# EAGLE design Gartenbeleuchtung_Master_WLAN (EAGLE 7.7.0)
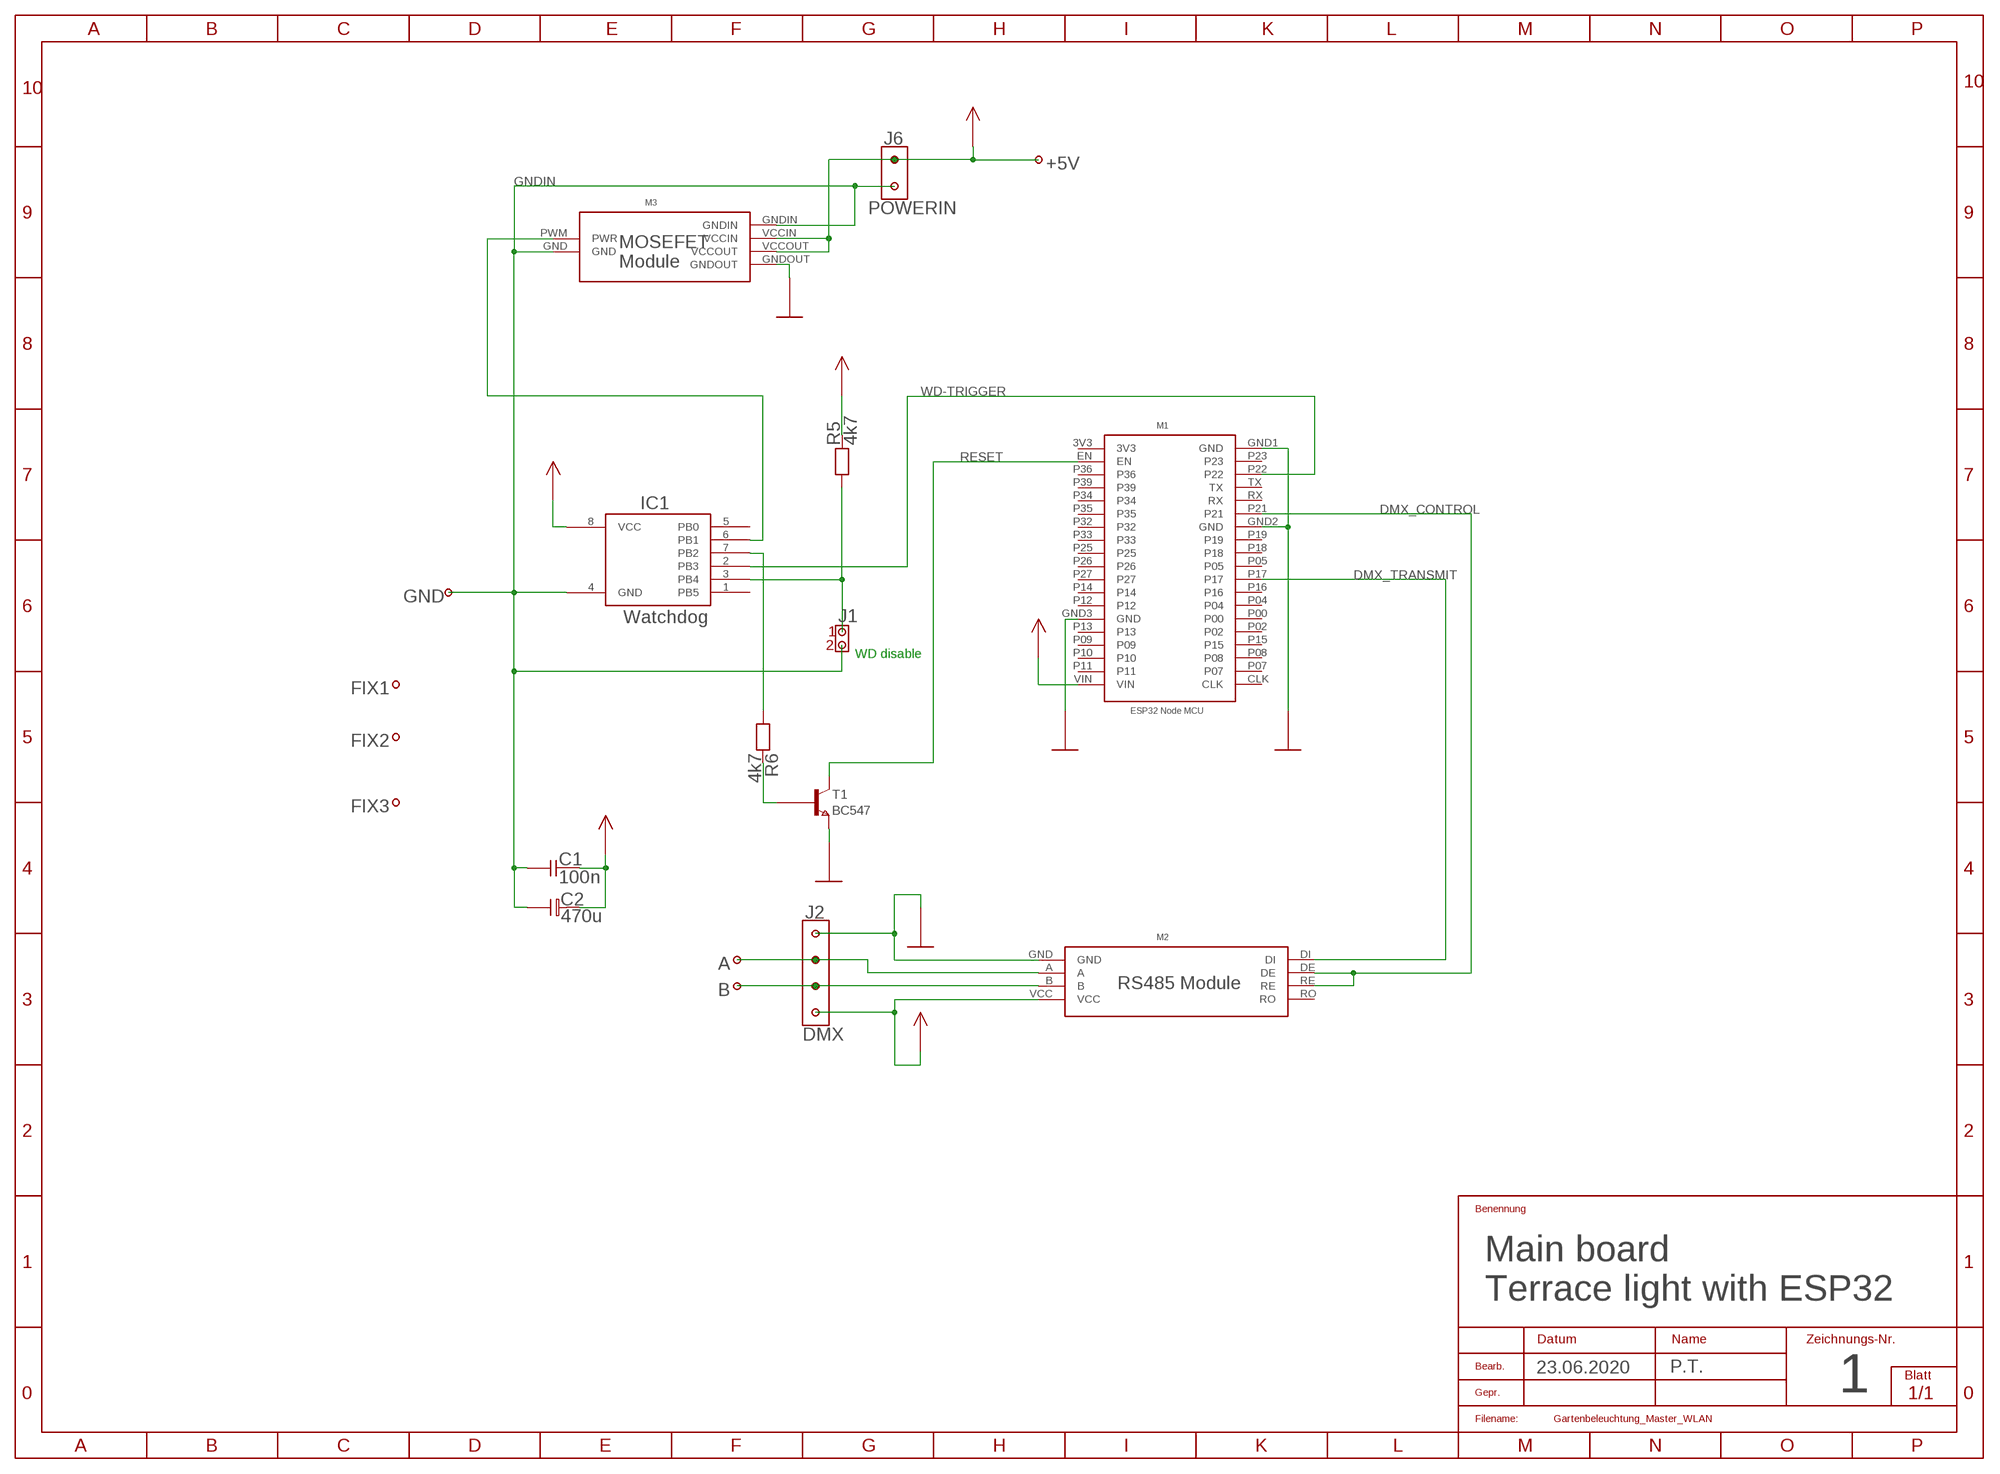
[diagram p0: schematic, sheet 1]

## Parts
+5V  PIN  [PIN]
A  PIN  [PIN]
B  PIN  [PIN]
C1  100n  CAP02  [CAP02B]
C2  470u  ELK02LI  [ELKOL02B]
FIX1  PIN  [PIN]
FIX2  PIN  [PIN]
FIX3  PIN  [PIN]
GND  PIN  [PIN]
IC1  Watchdog  ATINY13A  [DIL8]
J1  WD disable  CON02X1  [CON02X1]
J2  DMX  POWER4X1  [POWER4X1]
J6  POWERIN  POWER2X1  [POWER2X1]
M1  ESP32-NODEMCU1  [ESP32-NODEMCU1]
M2  RS485  [RS485]
M3  MOSFET  [MOSFET]
R5  4k7  RES04  [RES04B]
R6  4k7  RES04  [RES04B]
T1  BC547  BC237  [TO92A]

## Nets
DMX_CONTROL: M1.P21 M2.DE M2.RE
DMX_TRANSMIT: M1.P17 M2.DI
GND: J2.4 M1.GND1(GND) M1.GND2(GND) M1.GND3(GND) M2.GND M3.GNDOUT T1.3(E)
GNDIN: C1.1 C2.N GND.1 IC1.4(GND) J1.2 J6.1 M3.GND M3.GNDIN
N$4: IC1.3(PB4) J1.1 R5.1
N$5: A.1 J2.3 M2.A
N$6: B.1 J2.2 M2.B
N$7: IC1.7(PB2) R6.1
N$8: IC1.6(PB1) M3.PWM(PWR)
N$9: R6.2 T1.2(B)
RESET: M1.EN T1.1(C)
VCC: +5V.1 C1.2 C2.P IC1.8(VCC) J2.1 J6.2 M1.VIN M2.VCC M3.VCCIN M3.VCCOUT R5.2
WD-TRIGGER: IC1.2(PB3) M1.P22
Unconnected: FIX1.1 FIX2.1 FIX3.1 IC1.1(PB5) IC1.5(PB0) M1.CLK M1.P00 M1.P02 M1.P04 M1.P05 M1.P07 M1.P08 M1.P09 M1.P10 M1.P11 M1.P12 M1.P13 M1.P14 M1.P15 M1.P16 M1.P18 M1.P19 M1.P23 M1.P25 M1.P26 M1.P27 M1.P32 M1.P33 M1.P34 M1.P35 M1.P36 M1.P39 M1.RX M1.TX M2.RO

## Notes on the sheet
- WD disable
- Main board
- Terrace light with ESP32
- 23.06.2020 | P.T.
- 1

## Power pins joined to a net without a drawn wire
3V3: M1.3V3

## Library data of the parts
+5V A B FIX1-FIX3 GND = Connector 2:PIN
C1 = Discrete:CAP02
C2 = Discrete:ELK02LI
IC1 = Processor:ATINY13A
J1 = Connector 1:CON02X1
J2 = Connector 2:POWER4X1
J6 = Connector 2:POWER2X1
M1 = Giess:ESP32-NODEMCU1
M2 = Giess:RS485
M3 = Giess:MOSFET
R5 R6 = Discrete:RES04
T1 = Transistor:BC237

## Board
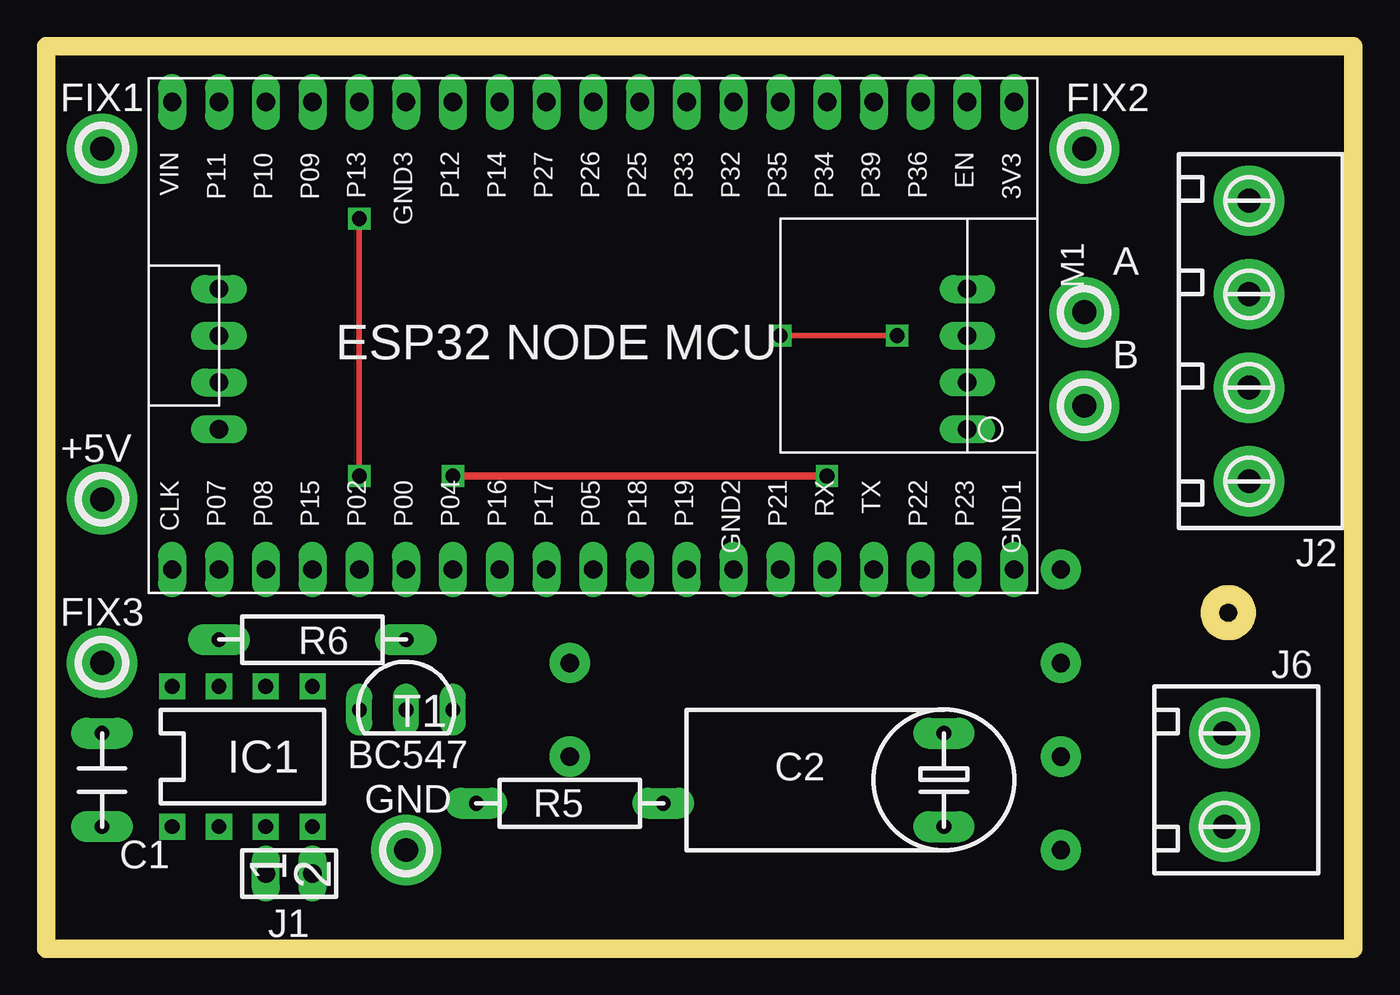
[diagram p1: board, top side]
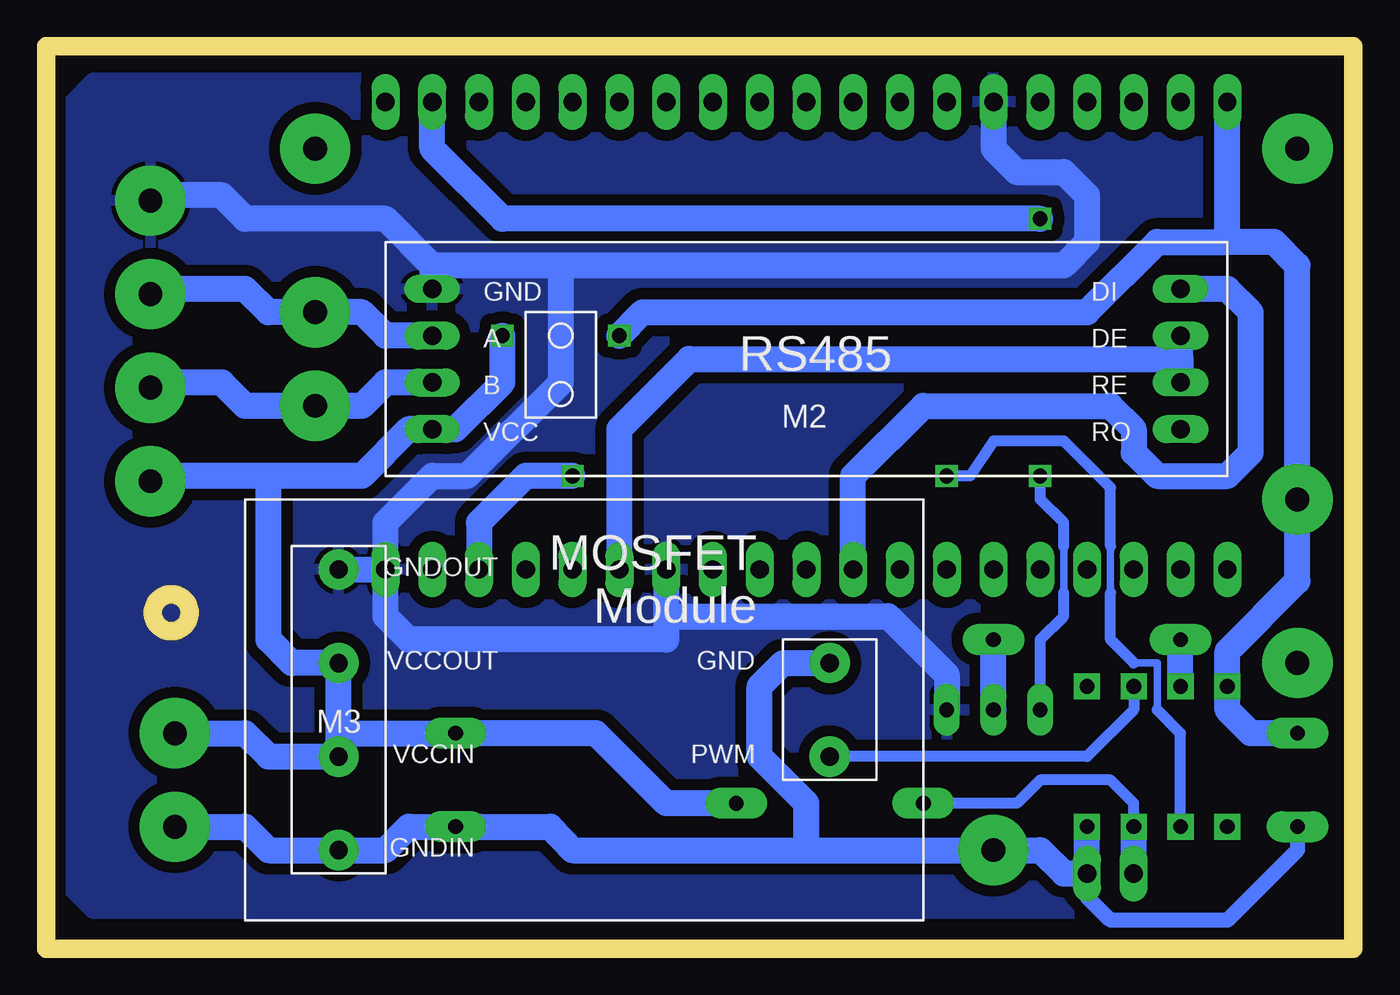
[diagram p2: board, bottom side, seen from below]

Size 71 x 49.04 mm. Coordinates in mm from the lower left corner, seen from the top.
Outline: 0,49.04 71,49.04 71,0 0,0 0,49.04
Copper layers (1*16): Top 0.035mm / dielectric 1.5mm / Bottom 0.035mm
Design rules "default": minimum track width 10mil, minimum drill 24mil, track to track 8mil, track to pad 8mil, pad to pad 8mil, via to via 8mil, smd to smd 8mil, copper to edge 40mil, drill to drill 8mil, minimum pad ring 10mil, minimum via ring 8mil, stop-mask expansion 4mil, vias tented up to drill 0mil, thermal gap 10mil
Milling: 6 lines

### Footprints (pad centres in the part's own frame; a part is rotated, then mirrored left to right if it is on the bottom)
PIN = drill 1.3 pad 3.81: 1 0,0
CAP02B = drill 0.8 pad 1.676 long: 1 0,0; 2 5.08,0
ELKOL02B = drill 0.8 pad 1.676 long: N 5.08,0; P 0,0
DIL8 = drill 0.8 pad 1.422 square: 1 0,0; 2 2.54,0; 3 5.08,0; 4 7.62,0; 5 7.62,7.62; 6 5.08,7.62; 7 2.54,7.62; 8 0,7.62
CON02X1 = drill 1 pad 1.422 long: 1 0,0; 2 0,-2.54
POWER4X1 = drill 1.3 pad 3.81: 1 0,0; 2 0,5.08; 3 0,10.16; 4 0,15.24
POWER2X1 = drill 1.3 pad 3.81: 1 0,0; 2 0,5.08
ESP32-NODEMCU1 = drill 1 pad 1.422 long: 3V3 -22.86,-12.7; CLK 22.86,12.7; EN -20.32,-12.7; GND1 -22.86,12.7; GND2 -7.62,12.7; GND3 10.16,-12.7; P00 10.16,12.7; P02 12.7,12.7; P04 7.62,12.7; P05 0,12.7; P07 20.32,12.7; P08 17.78,12.7; P09 15.24,-12.7; P10 17.78,-12.7; P11 20.32,-12.7; P12 7.62,-12.7; P13 12.7,-12.7; P14 5.08,-12.7; P15 15.24,12.7; P16 5.08,12.7; P17 2.54,12.7; P18 -2.54,12.7; P19 -5.08,12.7; P21 -10.16,12.7; P22 -17.78,12.7; P23 -20.32,12.7; P25 -2.54,-12.7; P26 0,-12.7; P27 2.54,-12.7; P32 -7.62,-12.7; P33 -5.08,-12.7; P34 -12.7,-12.7; P35 -10.16,-12.7; P36 -17.78,-12.7; P39 -15.24,-12.7; RX -12.7,12.7; TX -15.24,12.7; VIN 22.86,-12.7
RS485 = drill 1 pad 1.422 long: A -20.32,0; B -20.32,-2.54; DE 20.32,0; DI 20.32,2.54; GND -20.32,2.54; RE 20.32,-2.54; RO 20.32,-5.08; VCC -20.32,-5.08
MOSFET = drill 1 pad 2.184: GND -19.05,-5.08; GNDIN 7.62,5.08; GNDOUT 7.62,-10.16; PWM -19.05,0; VCCIN 7.62,0; VCCOUT 7.62,-5.08
RES04B = drill 0.8 pad 1.676 long: 1 0,0; 2 10.16,0
TO92A = drill 0.8 pad 1.422 long: 1 0,0; 2 2.54,0; 3 5.08,0

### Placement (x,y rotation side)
+5V  3.04,24.42 0 top
A  56.38,34.58 0 top
B  56.38,29.5 0 top
C1  3.04,6.64 90 top
C2  48.76,11.72 270 top
FIX1  3.04,43.47 0 top
FIX2  56.38,43.47 0 top
FIX3  3.04,15.53 0 top
GND  19.55,5.37 0 top
IC1  6.85,6.64 0 top
J1  11.93,4.1 90 top
J2  65.33,25.4 0 top
J6  64,6.64 0 top
M1  29.71,33.31 180 top
M2  29.71,33.31 0 bottom
M3  47.49,10.45 180 bottom
R5  23.36,7.91 0 top
R6  9.39,16.8 0 top
T1  17.01,12.99 0 top

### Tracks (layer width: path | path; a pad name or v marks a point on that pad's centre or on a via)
DMX_CONTROL
  Bottom 1.422: M1.P21 39.87,28.23 36.06,32.04 9.39,32.04 | 9.39,32.04 M2.RE | 9.39,32.04 M2.DE
DMX_TRANSMIT
  Bottom 1.422: M1.P17 27.17,25.69 23.36,29.5 13.2,29.5 11.93,28.23 11.93,26.96 10.66,25.69 6.85,25.69 5.58,26.96 5.58,34.58 6.85,35.85 M2.DI
GND
  Bottom 1.422: M3.GNDOUT M1.GND1 | 37.33,18.07 37.33,16.8 51.3,16.8 52.57,18.07 M1.GND1 | M1.GND2 37.33,18.07 | 37.33,18.07 25.27,18.07 22.09,14.9 T1.3 | M1.GND3 19.55,43.47 18.28,42.2 15.74,42.2 14.47,40.93 14.47,38.39 15.74,37.12 43.05,37.12 | 50.03,37.12 52.57,39.66 60.19,39.66 61.46,40.93 65.04,40.93 J2.4 | M1.GND1 52.57,23.15 50.03,25.69 48.12,25.69 43.05,30.77 43.05,37.12 | 43.05,37.12 50.03,37.12 | 50.03,37.12 M2.GND
  pour Bottom (isolate 0.61): 5.83,47.28 68.51,47.28 69.84,45.95 69.84,3.27 68.51,1.94 1.83,1.94 0.5,3.27 0.5,45.95 1.83,47.28
GNDIN
  Bottom 0.813: C1.1 3.04,5.37 6.85,1.56 13.2,1.56 14.47,2.83 J1.2
  Bottom 1.422: J6.1 60.19,6.64 58.92,5.37 M3.GNDIN 52.57,5.37 51.3,6.64 C2.N | 47.49,6.64 C2.N | C2.N 43.62,6.64 42.41,5.37 29.71,5.37 | 29.71,5.37 29.71,7.91 32.25,10.45 32.25,14.26 30.98,15.53 M3.GND | IC1.4 J1.2 15.74,4.1 17.01,5.37 GND.1 29.71,5.37
N$4
  Bottom 0.61: IC1.3 11.93,7.91 13.2,9.18 17.01,9.18 18.28,7.91 R5.1
  Bottom 1.422: J1.1 IC1.3
N$5
  Bottom 1.422: M2.A 52.57,33.31 53.84,34.58 A.1 58.92,34.58 60.19,35.85 65.04,35.85 J2.3
N$6
  Bottom 1.422: M2.B 52.57,30.77 53.84,29.5 B.1 60.19,29.5 61.46,30.77 65.27,30.77 65.27,30.54 J2.2
N$7
  Bottom 1.422: IC1.7 R6.1
N$8
  Bottom 0.61: IC1.6 11.93,12.99 14.47,10.45 M3.PWM
N$9
  Bottom 1.422: T1.2 R6.2
RESET  (via drill 0.8 pad 0.61, 0.8 pad 0.81)
  Top 0.305: v17.01,25.69 v17.01,39.66
  Bottom 0.406: 15.74,19.34 15.74,21.88
  Bottom 0.61: T1.1 17.01,16.8 15.74,18.07 15.74,19.34 | 15.74,21.88 15.74,23.15 17.01,24.42 v17.01,25.69
  Bottom 1.422: v17.01,39.66 46.22,39.66 50.03,43.47 M1.EN
VCC  (via drill 0.8 pad 0.81)
  Top 0.305: v46.22,33.31 v39.87,33.31
  Bottom 1.422: J6.2 60.19,11.72 58.92,10.45 M3.VCCIN | M3.VCCIN M3.VCCOUT 57.65,15.53 58.92,16.8 58.92,25.69 | M3.VCCIN 55.11,11.72 C2.P 41.14,11.72 37.33,7.91 R5.2 | C1.2 5.58,11.72 6.85,12.99 IC1.8 6.85,16.17 3.04,19.98 +5V.1 3.04,37.12 4.31,38.39 6.85,38.39 | 65.62,25.69 J2.1 65.04,25.69 58.92,25.69 | 58.92,25.69 53.84,25.69 51.3,28.23 M2.VCC 48.76,28.23 46.22,30.77 v46.22,33.31 | 6.85,38.39 M1.VIN | v39.87,33.31 38.6,34.58 14.47,34.58 10.66,38.39 6.85,38.39
WD-TRIGGER  (via drill 0.8 pad 0.61)
  Top 0.406: v22.09,25.69 v42.41,25.69
  Bottom 0.406: 10.66,12.99 10.66,15.53 11.93,15.53 | 13.2,19.34 13.2,21.88
  Bottom 0.61: IC1.2 9.39,11.72 10.66,12.99 | 11.93,15.53 13.2,16.8 13.2,19.34 | 13.2,21.88 13.2,25.05 15.74,27.6 19.55,27.6 20.82,25.69 v22.09,25.69
  Bottom 1.422: v42.41,25.69 44.95,25.69 47.49,23.15 M1.P22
